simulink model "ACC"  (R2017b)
settings: Solver=FixedStepDiscrete  StartTime=0.0  StopTime=10.0  FixedStep=0.01  RelTol=1e-3  EnableMultiTasking=on
undefined symbols (not defined in the file): ACC_CONST0_NUMB, ACC_CONST1000_NUMB, ACC_CONST100_NUMB, ACC_CONST121_NUMB, ACC_CONST1_NUMB, ACC_CONST2047_NUMB, ACC_CONST60000_NUMB, ACC_CONST60_NUMB, ACC_CONSTF1_NUMB, ACC_RUNTIME_MS, ASWTYPE_FALSE, ASWTYPE_TRUE, CcACC_ACChrgDispSOCPrmt_pct, CcACC_ACChrgMismatch_ms, CcACC_ACChrgPACKVolLim_V, CcACC_ACChrgPACKVolLimTi_ms, CcACC_ACChrgPrmtObcFltLvl_numb, CcACC_ACChrgPrmtVcuFltLvl_numb, CcACC_ACChrgStepCurr_A, CcACC_ACChrgTempPrmtDelayTime_ms, CcACC_ACCrntUnctrolTi_ms, CcACC_ACFullChrgHysVolt_mV, CcACC_ACFullStepChrgTi1_ms, CcACC_ACFullStepChrgTi2_ms, CcACC_ACMaxChrgCurr_A, CcACC_ACStepChrgWaitTime_ms, CcACC_ACStop2DefaultTi_ms, CcACC_ACStop2DefaultTiDelay_ms, CcACC_BatFullResetTime_ms, CcACC_ChrgCrnt0HysVolt_mV, CcACC_ChrgEndDeviationVol1_mV, CcACC_ChrgEndDeviationVol2_mV, CcACC_ChrgEndDeviationVol3_mV, CcACC_ChrgMaxPackVoltLimt_V, CcACC_ChrgPwr1_W, CcACC_ChrgPwr2_W, CcACC_ChrgPwr3_W, CcACC_ChrgSt2StepChrgDeviVol_mV, CcACC_ChrgSt2StepChrgTime_ms, CcACC_ChrgStCutoffTime_ms, CcACC_ChrgStFullChrgCrnt_A, CcACC_CPDutyLowThrhd_pct, CcACC_CrntFilterTi1_cnt, CcACC_CrntFilterTi2_cnt, CcACC_CrntFilterTi2_ms, CcACC_CurrObcPreHeatLowThrhd_A, CcACC_DiffACChrgCrnt_A, CcACC_DiffACChrgCrntTi_ms, CcACC_DispSOCCalStart_pct, CcACC_DispSOCDiff_pct, CcACC_ElecLckRemTimeHold_ms, CcACC_HeatChrgCrnt0Time_ms, CcACC_HeatChrgCrnt1Time_ms, CcACC_Initial500Ti_ms, CcACC_Initial700Ti_ms, CcACC_MaxACChrgCellTemp_C, CcACC_MaxPackVoltLimt_V, CcACC_MinACChrgCellTemp_C, CcACC_MinACChrgCrntRqst_A, CcACC_OBCChrgPwr_W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
libraries: AIWAYS_Powertrain_BMS_lib x94, simulink x2
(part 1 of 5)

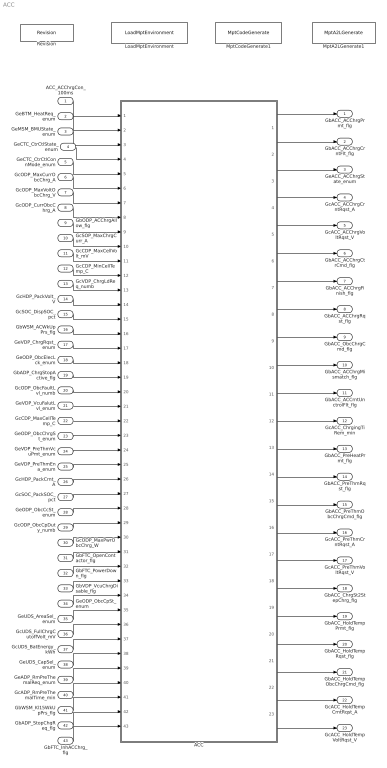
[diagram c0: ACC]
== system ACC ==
  ACC_ACChrgCon_100ms : Inport
  GeBTM_HeatReq_enum : Inport  Port=2
  GeMSM_BMUState_enum : Inport  Port=3
  GeCTC_CtrCtlState_enum : Inport  Port=4
  GeCTC_CtrCtlConnMode_enum : Inport  Port=5
  GcODP_MaxCurrObcChrg_A : Inport  Port=6
  GcODP_MaxVoltObcChrg_V : Inport  Port=7
  GcODP_CurrObcChrg_A : Inport  Port=8
  GbODP_ACChrgAllow_flg : Inport  Port=9
  GcSOP_MaxChrgCurr_A : Inport  Port=10
  GcCDP_MaxCellVolt_mV : Inport  Port=11
  GcCDP_MinCellTemp_C : Inport  Port=12
  GcVDP_ChrgLdReq_numb : Inport  Port=13
  GcHDP_PackVolt_V : Inport  Port=14
  GcSOC_DispSOC_pct : Inport  Port=15
  GbWSM_ACWkUpPrs_flg : Inport  Port=16
  GeVDP_ChrgRqst_enum : Inport  Port=17
  GeODP_ObcElecLck_enum : Inport  Port=18
  GbADP_ChrgStopActive_flg : Inport  Port=19
  GcODP_ObcFaultLvl_numb : Inport  Port=20
  GeVDP_VcuFalutLvl_enum : Inport  Port=21
  GcCDP_MaxCellTemp_C : Inport  Port=22
  GeODP_ObcChrgSt_enum : Inport  Port=23
  GeVDP_PreThmVcuPmt_enum : Inport  Port=24
  GeVDP_PreThmEna_enum : Inport  Port=25
  GcHDP_PackCrnt_A : Inport  Port=26
  GcSOC_PackSOC_pct : Inport  Port=27
  GeODP_ObcCcSt_enum : Inport  Port=28
  GcODP_ObcCpDuty_numb : Inport  Port=29
  GcODP_MaxPwrObcChrg_W : Inport  Port=30
  GbFTC_OpenContactor_flg : Inport  Port=31
  GbFTC_PowerDown_flg : Inport  Port=32
  GbVDP_VcuChrgDisable_flg : Inport  Port=33
  GeODP_ObcCpSt_enum : Inport  Port=34
  GeUDS_AreaSel_enum : Inport  Port=35
  GcUDS_FullChrgCutoffVolt_mV : Inport  Port=36
  GcUDS_BatEnergy_kWh : Inport  Port=37
  GeUDS_CapSel_enum : Inport  Port=38
  GeADP_RmPreThemalReq_enum : Inport  Port=39
  GcADP_RmPreThemalTime_min : Inport  Port=40
  GbWSM_Kl15WkUpPrs_flg : Inport  Port=41
  GbADP_StopChgReq_flg : Inport  Port=42
  GbFTC_InhACChrg_flg : Inport  Port=43
  ACC : Subsystem
  LoadMptEnvironment : AIWAYS_Powertrain_BMS_lib/Config/LoadMptEnvironment  ProjectName=Comm  SuppierID=NewPlatformUAES
  MptA2LGenerate1 : AIWAYS_Powertrain_BMS_lib/Config/MptA2LGenerate  SystemSampleTime=-1
  MptCodeGenerate1 : AIWAYS_Powertrain_BMS_lib/Config/MptCodeGenerate  SystemSampleTime=-1
  Revision : AIWAYS_Powertrain_BMS_lib/Config/Revision  curVersion='M106C108'  newVersion='M106C108'
  GbACC_ACChrgPrmt_flg : Outport
  GbACC_ACChrgCrntFlt_flg : Outport  Port=2
  GeACC_ACChrgState_enum : Outport  Port=3
  GcACC_ACChrgCrntRqst_A : Outport  Port=4
  GcACC_ACChrgVoltRqst_V : Outport  Port=5
  GbACC_ACChrgCtrCmd_flg : Outport  Port=6
  GbACC_ACChrgFinish_flg : Outport  Port=7
  GbACC_ACChrgRqst_flg : Outport  Port=8
  GbACC_ObcChrgCmd_flg : Outport  Port=9
  GbACC_ACChrgMismatch_flg : Outport  Port=10
  GbACC_ACCrntUnctrolFlt_flg : Outport  Port=11
  GcACC_ChrgingTiRem_min : Outport  Port=12
  GbACC_PreHeatPrmt_flg : Outport  Port=13
  GbACC_PreThmRqst_flg : Outport  Port=14
  GbACC_PreThmObcChrgCmd_flg : Outport  Port=15
  GcACC_PreThmCrntRqst_A : Outport  Port=16
  GcACC_PreThmVoltRqst_V : Outport  Port=17
  GbACC_ChrgSt2StepChrg_flg : Outport  Port=18
  GbACC_HoldTempPrmt_flg : Outport  Port=19
  GbACC_HoldTempRqst_flg : Outport  Port=20
  GbACC_HoldTempObcChrgCmd_flg : Outport  Port=21
  GcACC_HoldTempCrntRqst_A : Outport  Port=22
  GcACC_HoldTempVoltRqst_V : Outport  Port=23
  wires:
  ACC_ACChrgCon_100ms/1 -> ACC/1(ACC_ACChrgCon_100ms)
  GeBTM_HeatReq_enum/1 -> ACC/2(GeBTM_HeatReq_enum)
  GeMSM_BMUState_enum/1 -> ACC/3(GeMSM_BMUState_enum)
  GeCTC_CtrCtlState_enum/1 -> ACC/4(GeCTC_CtrCtlState_enum)
  GeCTC_CtrCtlConnMode_enum/1 -> ACC/5(GeCTC_CtrCtlConnMode_enum)
  GcODP_MaxCurrObcChrg_A/1 -> ACC/6(GcODP_MaxCurrObcChrg_A)
  GcODP_MaxVoltObcChrg_V/1 -> ACC/7(GcODP_MaxVoltObcChrg_V)
  GcODP_CurrObcChrg_A/1 -> ACC/8(GcODP_CurrObcChrg_A)
  GbODP_ACChrgAllow_flg/1 -> ACC/9(GbODP_ACChrgAllow_flg)
  GcSOP_MaxChrgCurr_A/1 -> ACC/10(GcSOP_MaxChrgCurr_A)
  GcCDP_MaxCellVolt_mV/1 -> ACC/11(GcCDP_MaxCellVolt_mV)
  GcCDP_MinCellTemp_C/1 -> ACC/12(GcCDP_MinCellTemp_C)
  GcVDP_ChrgLdReq_numb/1 -> ACC/13(GcVDP_ChrgLdReq_numb)
  GcHDP_PackVolt_V/1 -> ACC/14(GcHDP_PackVolt_V)
  GcSOC_DispSOC_pct/1 -> ACC/15(GcSOC_DispSOC_pct)
  GbWSM_ACWkUpPrs_flg/1 -> ACC/16(GbWSM_ACWkUpPrs_flg)
  GeVDP_ChrgRqst_enum/1 -> ACC/17(GeVDP_ChrgRqst_enum)
  GeODP_ObcElecLck_enum/1 -> ACC/18(GeODP_ObcElecLck_enum)
  ACC/1(GbACC_ACChrgPrmt_flg) -> GbACC_ACChrgPrmt_flg/1
  ACC/2(GbACC_ACChrgCrntFlt_flg) -> GbACC_ACChrgCrntFlt_flg/1
  ACC/3(GeACC_ACChrgState_enum) -> GeACC_ACChrgState_enum/1
  ACC/4(GcACC_ACChrgCrntRqst_A) -> GcACC_ACChrgCrntRqst_A/1
  ACC/5(GcACC_ACChrgVoltRqst_V) -> GcACC_ACChrgVoltRqst_V/1
  ACC/6(GbACC_ACChrgCtrCmd_flg) -> GbACC_ACChrgCtrCmd_flg/1
  ACC/7(GbACC_ACChrgFinish_flg) -> GbACC_ACChrgFinish_flg/1
  ACC/8(GbACC_ACChrgRqst_flg) -> GbACC_ACChrgRqst_flg/1
  ACC/9(GbACC_ObcChrgCmd_flg) -> GbACC_ObcChrgCmd_flg/1
  ACC/10(GbACC_ACChrgMismatch_flg) -> GbACC_ACChrgMismatch_flg/1
  ACC/11(GbACC_ACCrntUnctrolFlt_flg) -> GbACC_ACCrntUnctrolFlt_flg/1
  ACC/12(GcACC_ChrgingTiRem_min) -> GcACC_ChrgingTiRem_min/1
  GbADP_ChrgStopActive_flg/1 -> ACC/19(GbADP_ChrgStopActive_flg)
  GeODP_ObcChrgSt_enum/1 -> ACC/23(GeODP_ObcChrgSt_enum)
  GeVDP_VcuFalutLvl_enum/1 -> ACC/21(GeVDP_VcuFalutLvl_enum)
  GcODP_ObcFaultLvl_numb/1 -> ACC/20(GcODP_ObcFaultLvl_numb)
  GcCDP_MaxCellTemp_C/1 -> ACC/22(GcCDP_MaxCellTemp_C)
  ACC/13(GbACC_PreHeatPrmt_flg) -> GbACC_PreHeatPrmt_flg/1
  ACC/14(GbACC_PreThmRqst_flg) -> GbACC_PreThmRqst_flg/1
  GeVDP_PreThmVcuPmt_enum/1 -> ACC/24(GeVDP_PreThmVcuPmt_enum)
  GeVDP_PreThmEna_enum/1 -> ACC/25(GeVDP_PreThmEna_enum)
  ACC/15(GbACC_PreThmObcChrgCmd_flg) -> GbACC_PreThmObcChrgCmd_flg/1
  ACC/16(GcACC_PreThmCrntRqst_A) -> GcACC_PreThmCrntRqst_A/1
  ACC/17(GcACC_PreThmVoltRqst_V) -> GcACC_PreThmVoltRqst_V/1
  GcHDP_PackCrnt_A/1 -> ACC/26(GcHDP_PackCrnt_A)
  GcSOC_PackSOC_pct/1 -> ACC/27(GcSOC_PackSOC_pct)
  GeODP_ObcCcSt_enum/1 -> ACC/28(GeODP_ObcCcSt_enum)
  GcODP_ObcCpDuty_numb/1 -> ACC/29(GcODP_ObcCpDuty_numb)
  GcODP_MaxPwrObcChrg_W/1 -> ACC/30(GcODP_MaxPwrObcChrg_W)
  ACC/18(GbACC_ChrgSt2StepChrg_flg) -> GbACC_ChrgSt2StepChrg_flg/1
  GbFTC_OpenContactor_flg/1 -> ACC/31(GbFTC_OpenContactor_flg)
  GbFTC_PowerDown_flg/1 -> ACC/32(GbFTC_PowerDown_flg)
  GbVDP_VcuChrgDisable_flg/1 -> ACC/33(GbVDP_VcuChrgDisable_flg)
  GeODP_ObcCpSt_enum/1 -> ACC/34(GeODP_ObcCpSt_enum)
  GeUDS_AreaSel_enum/1 -> ACC/35(GeUDS_AreaSel_enum)
  GcUDS_FullChrgCutoffVolt_mV/1 -> ACC/36(GcUDS_FullChrgCutoffVolt_mV)
  GcUDS_BatEnergy_kWh/1 -> ACC/37(GcUDS_BatEnergy_kWh)
  GeUDS_CapSel_enum/1 -> ACC/38(GeUDS_CapSel_enum)
  GeADP_RmPreThemalReq_enum/1 -> ACC/39(GeADP_RmPreThemalReq_enum)
  GcADP_RmPreThemalTime_min/1 -> ACC/40(GcADP_RmPreThemalTime_min)
  GbWSM_Kl15WkUpPrs_flg/1 -> ACC/41(GbWSM_Kl15WkUpPrs_flg)
  ACC/19(GbACC_HoldTempPrmt_flg) -> GbACC_HoldTempPrmt_flg/1
  ACC/20(GbACC_HoldTempRqst_flg) -> GbACC_HoldTempRqst_flg/1
  ACC/21(GbACC_HoldTempObcChrgCmd_flg) -> GbACC_HoldTempObcChrgCmd_flg/1
  ACC/22(GcACC_HoldTempCrntRqst_A) -> GcACC_HoldTempCrntRqst_A/1
  ACC/23(GcACC_HoldTempVoltRqst_V) -> GcACC_HoldTempVoltRqst_V/1
  GbADP_StopChgReq_flg/1 -> ACC/42(GbADP_StopChgReq_flg)
  GbFTC_InhACChrg_flg/1 -> ACC/43(GbFTC_InhACChrg_flg)

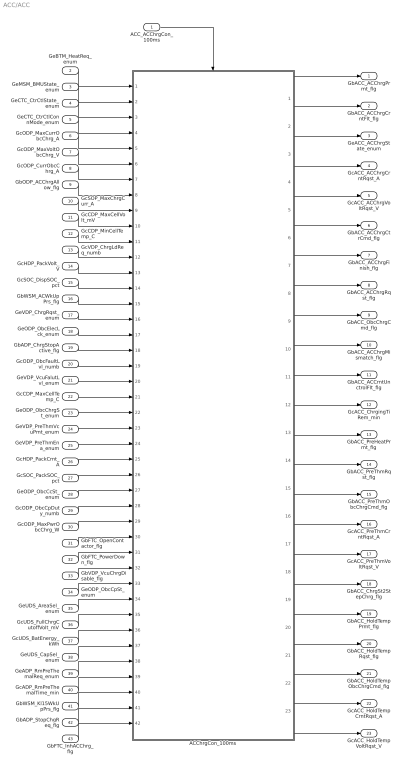
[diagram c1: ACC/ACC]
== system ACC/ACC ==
  ACC_ACChrgCon_100ms : Inport
  GeBTM_HeatReq_enum : Inport  Port=2
  GeMSM_BMUState_enum : Inport  Port=3
  GeCTC_CtrCtlState_enum : Inport  Port=4
  GeCTC_CtrCtlConnMode_enum : Inport  Port=5
  GcODP_MaxCurrObcChrg_A : Inport  Port=6
  GcODP_MaxVoltObcChrg_V : Inport  Port=7
  GcODP_CurrObcChrg_A : Inport  Port=8
  GbODP_ACChrgAllow_flg : Inport  Port=9
  GcSOP_MaxChrgCurr_A : Inport  Port=10
  GcCDP_MaxCellVolt_mV : Inport  Port=11
  GcCDP_MinCellTemp_C : Inport  Port=12
  GcVDP_ChrgLdReq_numb : Inport  Port=13
  GcHDP_PackVolt_V : Inport  Port=14
  GcSOC_DispSOC_pct : Inport  Port=15
  GbWSM_ACWkUpPrs_flg : Inport  Port=16
  GeVDP_ChrgRqst_enum : Inport  Port=17
  GeODP_ObcElecLck_enum : Inport  Port=18
  GbADP_ChrgStopActive_flg : Inport  Port=19
  GcODP_ObcFaultLvl_numb : Inport  Port=20
  GeVDP_VcuFalutLvl_enum : Inport  Port=21
  GcCDP_MaxCellTemp_C : Inport  Port=22
  GeODP_ObcChrgSt_enum : Inport  Port=23
  GeVDP_PreThmVcuPmt_enum : Inport  Port=24
  GeVDP_PreThmEna_enum : Inport  Port=25
  GcHDP_PackCrnt_A : Inport  Port=26
  GcSOC_PackSOC_pct : Inport  Port=27
  GeODP_ObcCcSt_enum : Inport  Port=28
  GcODP_ObcCpDuty_numb : Inport  Port=29
  GcODP_MaxPwrObcChrg_W : Inport  Port=30
  GbFTC_OpenContactor_flg : Inport  Port=31
  GbFTC_PowerDown_flg : Inport  Port=32
  GbVDP_VcuChrgDisable_flg : Inport  Port=33
  GeODP_ObcCpSt_enum : Inport  Port=34
  GeUDS_AreaSel_enum : Inport  Port=35
  GcUDS_FullChrgCutoffVolt_mV : Inport  Port=36
  GcUDS_BatEnergy_kWh : Inport  Port=37
  GeUDS_CapSel_enum : Inport  Port=38
  GeADP_RmPreThemalReq_enum : Inport  Port=39
  GcADP_RmPreThemalTime_min : Inport  Port=40
  GbWSM_Kl15WkUpPrs_flg : Inport  Port=41
  GbADP_StopChgReq_flg : Inport  Port=42
  GbFTC_InhACChrg_flg : Inport  Port=43
  ACChrgCon_100ms : Subsystem
  GbACC_ACChrgPrmt_flg : Outport
  GbACC_ACChrgCrntFlt_flg : Outport  Port=2
  GeACC_ACChrgState_enum : Outport  Port=3
  GcACC_ACChrgCrntRqst_A : Outport  Port=4
  GcACC_ACChrgVoltRqst_V : Outport  Port=5
  GbACC_ACChrgCtrCmd_flg : Outport  Port=6
  GbACC_ACChrgFinish_flg : Outport  Port=7
  GbACC_ACChrgRqst_flg : Outport  Port=8
  GbACC_ObcChrgCmd_flg : Outport  Port=9
  GbACC_ACChrgMismatch_flg : Outport  Port=10
  GbACC_ACCrntUnctrolFlt_flg : Outport  Port=11
  GcACC_ChrgingTiRem_min : Outport  Port=12
  GbACC_PreHeatPrmt_flg : Outport  Port=13
  GbACC_PreThmRqst_flg : Outport  Port=14
  GbACC_PreThmObcChrgCmd_flg : Outport  Port=15
  GcACC_PreThmCrntRqst_A : Outport  Port=16
  GcACC_PreThmVoltRqst_V : Outport  Port=17
  GbACC_ChrgSt2StepChrg_flg : Outport  Port=18
  GbACC_HoldTempPrmt_flg : Outport  Port=19
  GbACC_HoldTempRqst_flg : Outport  Port=20
  GbACC_HoldTempObcChrgCmd_flg : Outport  Port=21
  GcACC_HoldTempCrntRqst_A : Outport  Port=22
  GcACC_HoldTempVoltRqst_V : Outport  Port=23
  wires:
  ACC_ACChrgCon_100ms/1 -> ACChrgCon_100ms/Trigger
  GeBTM_HeatReq_enum/1 -> ACChrgCon_100ms/1(GeBTM_HeatReq_enum)
  GeMSM_BMUState_enum/1 -> ACChrgCon_100ms/2(GeMSM_BMUState_enum)
  GeCTC_CtrCtlState_enum/1 -> ACChrgCon_100ms/3(GeCTC_CtrCtlState_enum)
  GeCTC_CtrCtlConnMode_enum/1 -> ACChrgCon_100ms/4(GeCTC_CtrCtlConnMode_enum)
  GcODP_MaxCurrObcChrg_A/1 -> ACChrgCon_100ms/5(GcODP_MaxCurrObcChrg_A)
  GcODP_MaxVoltObcChrg_V/1 -> ACChrgCon_100ms/6(GcODP_MaxVoltObcChrg_V)
  GcODP_CurrObcChrg_A/1 -> ACChrgCon_100ms/7(GcODP_CurrObcChrg_A)
  GbODP_ACChrgAllow_flg/1 -> ACChrgCon_100ms/8(GbODP_ACChrgAllow_flg)
  GcSOP_MaxChrgCurr_A/1 -> ACChrgCon_100ms/9(GcSOP_MaxChrgCurr_A)
  GcCDP_MaxCellVolt_mV/1 -> ACChrgCon_100ms/10(GcCDP_MaxCellVolt_mV)
  GcCDP_MinCellTemp_C/1 -> ACChrgCon_100ms/11(GcCDP_MinCellTemp_C)
  GcVDP_ChrgLdReq_numb/1 -> ACChrgCon_100ms/12(GcVDP_ChrgLdReq_numb)
  GcHDP_PackVolt_V/1 -> ACChrgCon_100ms/13(GcHDP_PackVolt_V)
  GcSOC_DispSOC_pct/1 -> ACChrgCon_100ms/14(GcSOC_DispSOC_pct)
  GbWSM_ACWkUpPrs_flg/1 -> ACChrgCon_100ms/15(GbWSM_ACWkUpPrs_flg)
  GeVDP_ChrgRqst_enum/1 -> ACChrgCon_100ms/16(GeVDP_ChrgRqst_enum)
  GeODP_ObcElecLck_enum/1 -> ACChrgCon_100ms/17(GeODP_ObcElecLck_enum)
  ACChrgCon_100ms/1(GbACC_ACChrgPrmt_flg) -> GbACC_ACChrgPrmt_flg/1
  ACChrgCon_100ms/2(GbACC_ACChrgCrntFlt_flg) -> GbACC_ACChrgCrntFlt_flg/1
  ACChrgCon_100ms/3(GeACC_ACChrgState_enum) -> GeACC_ACChrgState_enum/1
  ACChrgCon_100ms/4(GcACC_ACChrgCrntRqst_A) -> GcACC_ACChrgCrntRqst_A/1
  ACChrgCon_100ms/5(GcACC_ACChrgVoltRqst_V) -> GcACC_ACChrgVoltRqst_V/1
  ACChrgCon_100ms/6(GbACC_ACChrgCtrCmd_flg) -> GbACC_ACChrgCtrCmd_flg/1
  ACChrgCon_100ms/7(GbACC_ACChrgFinish_flg) -> GbACC_ACChrgFinish_flg/1
  ACChrgCon_100ms/8(GbACC_ACChrgRqst_flg) -> GbACC_ACChrgRqst_flg/1
  ACChrgCon_100ms/9(GbACC_ObcChrgCmd_flg) -> GbACC_ObcChrgCmd_flg/1
  ACChrgCon_100ms/10(GbACC_ACChrgMismatch_flg) -> GbACC_ACChrgMismatch_flg/1
  ACChrgCon_100ms/11(GbACC_ACCrntUnctrolFlt_flg) -> GbACC_ACCrntUnctrolFlt_flg/1
  ACChrgCon_100ms/12(GcACC_ChrgingTiRem_min) -> GcACC_ChrgingTiRem_min/1
  GbADP_ChrgStopActive_flg/1 -> ACChrgCon_100ms/18(GbADP_ChrgStopActive_flg)
  GcODP_ObcFaultLvl_numb/1 -> ACChrgCon_100ms/19(GcODP_ObcFaultLvl_numb)
  GeVDP_VcuFalutLvl_enum/1 -> ACChrgCon_100ms/20(GeVDP_VcuFalutLvl_enum)
  GcCDP_MaxCellTemp_C/1 -> ACChrgCon_100ms/21(GcCDP_MaxCellTemp_C)
  GeODP_ObcChrgSt_enum/1 -> ACChrgCon_100ms/22(GeODP_ObcChrgSt_enum)
  GeVDP_PreThmVcuPmt_enum/1 -> ACChrgCon_100ms/23(GeVDP_PreThmVcuPmt_enum)
  GeVDP_PreThmEna_enum/1 -> ACChrgCon_100ms/24(GeVDP_PreThmEna_enum)
  ACChrgCon_100ms/13(GbACC_PreHeatPrmt_flg) -> GbACC_PreHeatPrmt_flg/1
  ACChrgCon_100ms/14(GbACC_PreThmRqst_flg) -> GbACC_PreThmRqst_flg/1
  ACChrgCon_100ms/15(GbACC_PreThmObcChrgCmd_flg) -> GbACC_PreThmObcChrgCmd_flg/1
  ACChrgCon_100ms/16(GcACC_PreThmCrntRqst_A) -> GcACC_PreThmCrntRqst_A/1
  ACChrgCon_100ms/17(GcACC_PreThmVoltRqst_V) -> GcACC_PreThmVoltRqst_V/1
  GcHDP_PackCrnt_A/1 -> ACChrgCon_100ms/25(GcHDP_PackCrnt_A)
  GcSOC_PackSOC_pct/1 -> ACChrgCon_100ms/26(GcSOC_PackSOC_pct)
  GeODP_ObcCcSt_enum/1 -> ACChrgCon_100ms/27(GeODP_ObcCcSt_enum)
  GcODP_ObcCpDuty_numb/1 -> ACChrgCon_100ms/28(GcODP_ObcCpDuty_numb)
  GcODP_MaxPwrObcChrg_W/1 -> ACChrgCon_100ms/29(GcODP_MaxPwrObcChrg_W)
  ACChrgCon_100ms/18(GbACC_ChrgSt2StepChrg_flg) -> GbACC_ChrgSt2StepChrg_flg/1
  GbFTC_OpenContactor_flg/1 -> ACChrgCon_100ms/30(GbFTC_OpenContactor_flg)
  GbFTC_PowerDown_flg/1 -> ACChrgCon_100ms/31(GbFTC_PowerDown_flg)
  GbVDP_VcuChrgDisable_flg/1 -> ACChrgCon_100ms/32(GbVDP_VcuChrgDisable_flg)
  GeODP_ObcCpSt_enum/1 -> ACChrgCon_100ms/33(GeODP_ObcCpSt_enum)
  GeUDS_AreaSel_enum/1 -> ACChrgCon_100ms/34(GeUDS_AreaSel_enum)
  GcUDS_FullChrgCutoffVolt_mV/1 -> ACChrgCon_100ms/35(GcUDS_FullChrgCutoffVolt_mV)
  GcUDS_BatEnergy_kWh/1 -> ACChrgCon_100ms/36(GcUDS_BatEnergy_kWh)
  GeUDS_CapSel_enum/1 -> ACChrgCon_100ms/37(GeUDS_CapSel_enum)
  ACChrgCon_100ms/19(GbACC_HoldTempPrmt_flg) -> GbACC_HoldTempPrmt_flg/1
  ACChrgCon_100ms/20(GbACC_HoldTempRqst_flg) -> GbACC_HoldTempRqst_flg/1
  ACChrgCon_100ms/21(GbACC_HoldTempObcChrgCmd_flg) -> GbACC_HoldTempObcChrgCmd_flg/1
  ACChrgCon_100ms/22(GcACC_HoldTempCrntRqst_A) -> GcACC_HoldTempCrntRqst_A/1
  ACChrgCon_100ms/23(GcACC_HoldTempVoltRqst_V) -> GcACC_HoldTempVoltRqst_V/1
  GeADP_RmPreThemalReq_enum/1 -> ACChrgCon_100ms/38(GeADP_RmPreThemalReq_enum)
  GcADP_RmPreThemalTime_min/1 -> ACChrgCon_100ms/39(GcADP_RmPreThemalTime_min)
  GbWSM_Kl15WkUpPrs_flg/1 -> ACChrgCon_100ms/40(GbWSM_Kl15WkUpPrs_flg)
  GbADP_StopChgReq_flg/1 -> ACChrgCon_100ms/41(GbADP_StopChgReq_flg)
  GbFTC_InhACChrg_flg/1 -> ACChrgCon_100ms/42(GbFTC_InhACChrg_flg)

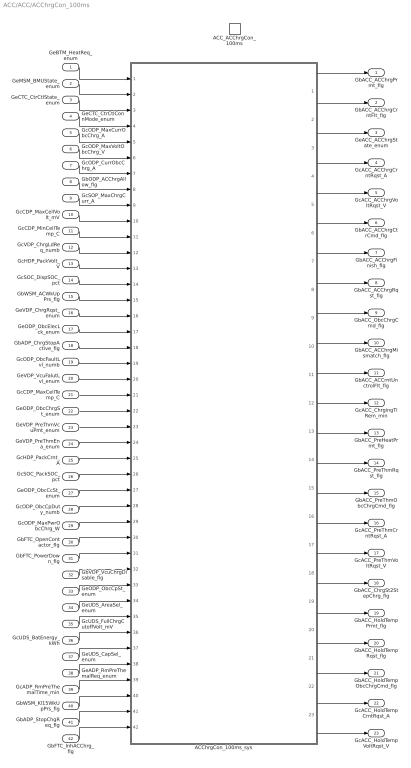
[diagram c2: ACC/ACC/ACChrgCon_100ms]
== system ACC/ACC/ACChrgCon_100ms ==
  GeBTM_HeatReq_enum : Inport
  GeMSM_BMUState_enum : Inport  Port=2
  GeCTC_CtrCtlState_enum : Inport  Port=3
  GeCTC_CtrCtlConnMode_enum : Inport  Port=4
  GcODP_MaxCurrObcChrg_A : Inport  Port=5
  GcODP_MaxVoltObcChrg_V : Inport  Port=6
  GcODP_CurrObcChrg_A : Inport  Port=7
  GbODP_ACChrgAllow_flg : Inport  Port=8
  GcSOP_MaxChrgCurr_A : Inport  Port=9
  GcCDP_MaxCellVolt_mV : Inport  Port=10
  GcCDP_MinCellTemp_C : Inport  Port=11
  GcVDP_ChrgLdReq_numb : Inport  Port=12
  GcHDP_PackVolt_V : Inport  Port=13
  GcSOC_DispSOC_pct : Inport  Port=14
  GbWSM_ACWkUpPrs_flg : Inport  Port=15
  GeVDP_ChrgRqst_enum : Inport  Port=16
  GeODP_ObcElecLck_enum : Inport  Port=17
  GbADP_ChrgStopActive_flg : Inport  Port=18
  GcODP_ObcFaultLvl_numb : Inport  Port=19
  GeVDP_VcuFalutLvl_enum : Inport  Port=20
  GcCDP_MaxCellTemp_C : Inport  Port=21
  GeODP_ObcChrgSt_enum : Inport  Port=22
  GeVDP_PreThmVcuPmt_enum : Inport  Port=23
  GeVDP_PreThmEna_enum : Inport  Port=24
  GcHDP_PackCrnt_A : Inport  Port=25
  GcSOC_PackSOC_pct : Inport  Port=26
  GeODP_ObcCcSt_enum : Inport  Port=27
  GcODP_ObcCpDuty_numb : Inport  Port=28
  GcODP_MaxPwrObcChrg_W : Inport  Port=29
  GbFTC_OpenContactor_flg : Inport  Port=30
  GbFTC_PowerDown_flg : Inport  Port=31
  GbVDP_VcuChrgDisable_flg : Inport  Port=32
  GeODP_ObcCpSt_enum : Inport  Port=33
  GeUDS_AreaSel_enum : Inport  Port=34
  GcUDS_FullChrgCutoffVolt_mV : Inport  Port=35
  GcUDS_BatEnergy_kWh : Inport  Port=36
  GeUDS_CapSel_enum : Inport  Port=37
  GeADP_RmPreThemalReq_enum : Inport  Port=38
  GcADP_RmPreThemalTime_min : Inport  Port=39
  GbWSM_Kl15WkUpPrs_flg : Inport  Port=40
  GbADP_StopChgReq_flg : Inport  Port=41
  GbFTC_InhACChrg_flg : Inport  Port=42
  ACC_ACChrgCon_100ms : TriggerPort  TriggerType=function-call  VariantControl=(inherit)
  ACChrgCon_100ms_sys : Subsystem
  GbACC_ACChrgPrmt_flg : Outport
  GbACC_ACChrgCrntFlt_flg : Outport  Port=2
  GeACC_ACChrgState_enum : Outport  Port=3
  GcACC_ACChrgCrntRqst_A : Outport  Port=4
  GcACC_ACChrgVoltRqst_V : Outport  Port=5
  GbACC_ACChrgCtrCmd_flg : Outport  Port=6
  GbACC_ACChrgFinish_flg : Outport  Port=7
  GbACC_ACChrgRqst_flg : Outport  Port=8
  GbACC_ObcChrgCmd_flg : Outport  Port=9
  GbACC_ACChrgMismatch_flg : Outport  Port=10
  GbACC_ACCrntUnctrolFlt_flg : Outport  Port=11
  GcACC_ChrgingTiRem_min : Outport  Port=12
  GbACC_PreHeatPrmt_flg : Outport  Port=13
  GbACC_PreThmRqst_flg : Outport  Port=14
  GbACC_PreThmObcChrgCmd_flg : Outport  Port=15
  GcACC_PreThmCrntRqst_A : Outport  Port=16
  GcACC_PreThmVoltRqst_V : Outport  Port=17
  GbACC_ChrgSt2StepChrg_flg : Outport  Port=18
  GbACC_HoldTempPrmt_flg : Outport  Port=19
  GbACC_HoldTempRqst_flg : Outport  Port=20
  GbACC_HoldTempObcChrgCmd_flg : Outport  Port=21
  GcACC_HoldTempCrntRqst_A : Outport  Port=22
  GcACC_HoldTempVoltRqst_V : Outport  Port=23
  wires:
  GeBTM_HeatReq_enum/1 -> ACChrgCon_100ms_sys/1(GeBTM_HeatReq_enum)
  GeMSM_BMUState_enum/1 -> ACChrgCon_100ms_sys/2(GeMSM_BMUState_enum)
  GeCTC_CtrCtlState_enum/1 -> ACChrgCon_100ms_sys/3(GeCTC_CtrCtlState_enum)
  GeCTC_CtrCtlConnMode_enum/1 -> ACChrgCon_100ms_sys/4(GeCTC_CtrCtlConnMode_enum)
  GcODP_MaxCurrObcChrg_A/1 -> ACChrgCon_100ms_sys/5(GcODP_MaxCurrObcChrg_A)
  GcODP_MaxVoltObcChrg_V/1 -> ACChrgCon_100ms_sys/6(GcODP_MaxVoltObcChrg_V)
  GcODP_CurrObcChrg_A/1 -> ACChrgCon_100ms_sys/7(GcODP_CurrObcChrg_A)
  GbODP_ACChrgAllow_flg/1 -> ACChrgCon_100ms_sys/8(GbODP_ACChrgAllow_flg)
  GcSOP_MaxChrgCurr_A/1 -> ACChrgCon_100ms_sys/9(GcSOP_MaxChrgCurr_A)
  GcCDP_MaxCellVolt_mV/1 -> ACChrgCon_100ms_sys/10(GcCDP_MaxCellVolt_mV)
  GcCDP_MinCellTemp_C/1 -> ACChrgCon_100ms_sys/11(GcCDP_MinCellTemp_C)
  GcVDP_ChrgLdReq_numb/1 -> ACChrgCon_100ms_sys/12(GcVDP_ChrgLdReq_numb)
  GcHDP_PackVolt_V/1 -> ACChrgCon_100ms_sys/13(GcHDP_PackVolt_V)
  GcSOC_DispSOC_pct/1 -> ACChrgCon_100ms_sys/14(GcSOC_DispSOC_pct)
  GbWSM_ACWkUpPrs_flg/1 -> ACChrgCon_100ms_sys/15(GbWSM_ACWkUpPrs_flg)
  GeVDP_ChrgRqst_enum/1 -> ACChrgCon_100ms_sys/16(GeVDP_ChrgRqst_enum)
  GeODP_ObcElecLck_enum/1 -> ACChrgCon_100ms_sys/17(GeODP_ObcElecLck_enum)
  ACChrgCon_100ms_sys/1(GbACC_ACChrgPrmt_flg) -> GbACC_ACChrgPrmt_flg/1
  ACChrgCon_100ms_sys/2(GbACC_ACChrgCrntFlt_flg) -> GbACC_ACChrgCrntFlt_flg/1
  ACChrgCon_100ms_sys/3(GeACC_ACChrgState_enum) -> GeACC_ACChrgState_enum/1
  ACChrgCon_100ms_sys/4(GcACC_ACChrgCrntRqst_A) -> GcACC_ACChrgCrntRqst_A/1
  ACChrgCon_100ms_sys/5(GcACC_ACChrgVoltRqst_V) -> GcACC_ACChrgVoltRqst_V/1
  ACChrgCon_100ms_sys/6(GbACC_ACChrgCtrCmd_flg) -> GbACC_ACChrgCtrCmd_flg/1
  ACChrgCon_100ms_sys/7(GbACC_ACChrgFinish_flg) -> GbACC_ACChrgFinish_flg/1
  ACChrgCon_100ms_sys/8(GbACC_ACChrgRqst_flg) -> GbACC_ACChrgRqst_flg/1
  ACChrgCon_100ms_sys/9(GbACC_ObcChrgCmd_flg) -> GbACC_ObcChrgCmd_flg/1
  ACChrgCon_100ms_sys/10(GbACC_ACChrgMismatch_flg) -> GbACC_ACChrgMismatch_flg/1
  ACChrgCon_100ms_sys/11(GbACC_ACCrntUnctrolFlt_flg) -> GbACC_ACCrntUnctrolFlt_flg/1
  ACChrgCon_100ms_sys/12(GcACC_ChrgingTiRem_min) -> GcACC_ChrgingTiRem_min/1
  GbADP_ChrgStopActive_flg/1 -> ACChrgCon_100ms_sys/18(GbADP_ChrgStopActive_flg)
  GcODP_ObcFaultLvl_numb/1 -> ACChrgCon_100ms_sys/19(GcODP_ObcFaultLvl_numb)
  GeVDP_VcuFalutLvl_enum/1 -> ACChrgCon_100ms_sys/20(GeVDP_VcuFalutLvl_enum)
  GcCDP_MaxCellTemp_C/1 -> ACChrgCon_100ms_sys/21(GcCDP_MaxCellTemp_C)
  GeODP_ObcChrgSt_enum/1 -> ACChrgCon_100ms_sys/22(GeODP_ObcChrgSt_enum)
  GeVDP_PreThmVcuPmt_enum/1 -> ACChrgCon_100ms_sys/23(GeVDP_PreThmVcuPmt_enum)
  GeVDP_PreThmEna_enum/1 -> ACChrgCon_100ms_sys/24(GeVDP_PreThmEna_enum)
  ACChrgCon_100ms_sys/13(GbACC_PreHeatPrmt_flg) -> GbACC_PreHeatPrmt_flg/1
  ACChrgCon_100ms_sys/14(GbACC_PreThmRqst_flg) -> GbACC_PreThmRqst_flg/1
  ACChrgCon_100ms_sys/15(GbACC_PreThmObcChrgCmd_flg) -> GbACC_PreThmObcChrgCmd_flg/1
  ACChrgCon_100ms_sys/16(GcACC_PreThmCrntRqst_A) -> GcACC_PreThmCrntRqst_A/1
  ACChrgCon_100ms_sys/17(GcACC_PreThmVoltRqst_V) -> GcACC_PreThmVoltRqst_V/1
  GcHDP_PackCrnt_A/1 -> ACChrgCon_100ms_sys/25(GcHDP_PackCrnt_A)
  GcSOC_PackSOC_pct/1 -> ACChrgCon_100ms_sys/26(GcSOC_PackSOC_pct)
  GeODP_ObcCcSt_enum/1 -> ACChrgCon_100ms_sys/27(GeODP_ObcCcSt_enum)
  GcODP_ObcCpDuty_numb/1 -> ACChrgCon_100ms_sys/28(GcODP_ObcCpDuty_numb)
  GcODP_MaxPwrObcChrg_W/1 -> ACChrgCon_100ms_sys/29(GcODP_MaxPwrObcChrg_W)
  ACChrgCon_100ms_sys/18(GbACC_ChrgSt2StepChrg_flg) -> GbACC_ChrgSt2StepChrg_flg/1
  GbFTC_OpenContactor_flg/1 -> ACChrgCon_100ms_sys/30(GbFTC_OpenContactor_flg)
  GbFTC_PowerDown_flg/1 -> ACChrgCon_100ms_sys/31(GbFTC_PowerDown_flg)
  GbVDP_VcuChrgDisable_flg/1 -> ACChrgCon_100ms_sys/32(GbVDP_VcuChrgDisable_flg)
  GeODP_ObcCpSt_enum/1 -> ACChrgCon_100ms_sys/33(GeODP_ObcCpSt_enum)
  GeUDS_AreaSel_enum/1 -> ACChrgCon_100ms_sys/34(GeUDS_AreaSel_enum)
  GcUDS_FullChrgCutoffVolt_mV/1 -> ACChrgCon_100ms_sys/35(GcUDS_FullChrgCutoffVolt_mV)
  GcUDS_BatEnergy_kWh/1 -> ACChrgCon_100ms_sys/36(GcUDS_BatEnergy_kWh)
  GeUDS_CapSel_enum/1 -> ACChrgCon_100ms_sys/37(GeUDS_CapSel_enum)
  GeADP_RmPreThemalReq_enum/1 -> ACChrgCon_100ms_sys/38(GeADP_RmPreThemalReq_enum)
  GcADP_RmPreThemalTime_min/1 -> ACChrgCon_100ms_sys/39(GcADP_RmPreThemalTime_min)
  GbWSM_Kl15WkUpPrs_flg/1 -> ACChrgCon_100ms_sys/40(GbWSM_Kl15WkUpPrs_flg)
  ACChrgCon_100ms_sys/19(GbACC_HoldTempPrmt_flg) -> GbACC_HoldTempPrmt_flg/1
  ACChrgCon_100ms_sys/20(GbACC_HoldTempRqst_flg) -> GbACC_HoldTempRqst_flg/1
  ACChrgCon_100ms_sys/21(GbACC_HoldTempObcChrgCmd_flg) -> GbACC_HoldTempObcChrgCmd_flg/1
  ACChrgCon_100ms_sys/22(GcACC_HoldTempCrntRqst_A) -> GcACC_HoldTempCrntRqst_A/1
  ACChrgCon_100ms_sys/23(GcACC_HoldTempVoltRqst_V) -> GcACC_HoldTempVoltRqst_V/1
  GbADP_StopChgReq_flg/1 -> ACChrgCon_100ms_sys/41(GbADP_StopChgReq_flg)
  GbFTC_InhACChrg_flg/1 -> ACChrgCon_100ms_sys/42(GbFTC_InhACChrg_flg)

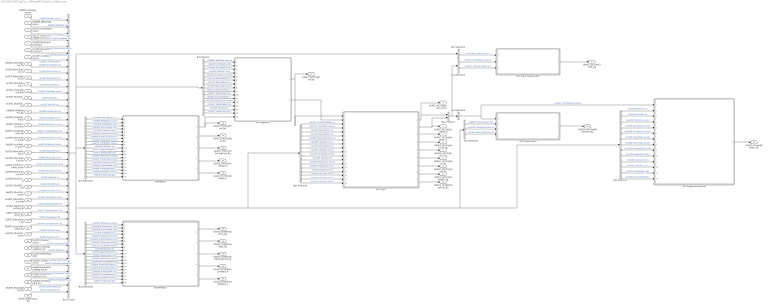
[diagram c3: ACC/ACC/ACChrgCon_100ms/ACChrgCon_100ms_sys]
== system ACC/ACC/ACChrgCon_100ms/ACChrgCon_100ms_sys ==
  GeBTM_HeatReq_enum : Inport
  GeMSM_BMUState_enum : Inport  Port=2
  GeCTC_CtrCtlState_enum : Inport  Port=3
  GeCTC_CtrCtlConnMode_enum : Inport  Port=4
  GcODP_MaxCurrObcChrg_A : Inport  Port=5
  GcODP_MaxVoltObcChrg_V : Inport  Port=6
  GcODP_CurrObcChrg_A : Inport  Port=7
  GbODP_ACChrgAllow_flg : Inport  Port=8
  GcSOP_MaxChrgCurr_A : Inport  Port=9
  GcCDP_MaxCellVolt_mV : Inport  Port=10
  GcCDP_MinCellTemp_C : Inport  Port=11
  GcVDP_ChrgLdReq_numb : Inport  Port=12
  GcHDP_PackVolt_V : Inport  Port=13
  GcSOC_DispSOC_pct : Inport  Port=14
  GbWSM_ACWkUpPrs_flg : Inport  Port=15
  GeVDP_ChrgRqst_enum : Inport  Port=16
  GeODP_ObcElecLck_enum : Inport  Port=17
  GbADP_ChrgStopActive_flg : Inport  Port=18
  GcODP_ObcFaultLvl_numb : Inport  Port=19
  GeVDP_VcuFalutLvl_enum : Inport  Port=20
  GcCDP_MaxCellTemp_C : Inport  Port=21
  GeODP_ObcChrgSt_enum : Inport  Port=22
  GeVDP_PreThmVcuPmt_enum : Inport  Port=23
  GeVDP_PreThmEna_enum : Inport  Port=24
  GcHDP_PackCrnt_A : Inport  Port=25
  GcSOC_PackSOC_pct : Inport  Port=26
  GeODP_ObcCcSt_enum : Inport  Port=27
  GcODP_ObcCpDuty_numb : Inport  Port=28
  GcODP_MaxPwrObcChrg_W : Inport  Port=29
  GbFTC_OpenContactor_flg : Inport  Port=30
  GbFTC_PowerDown_flg : Inport  Port=31
  GbVDP_VcuChrgDisable_flg : Inport  Port=32
  GeODP_ObcCpSt_enum : Inport  Port=33
  GeUDS_AreaSel_enum : Inport  Port=34
  GcUDS_FullChrgCutoffVolt_mV : Inport  Port=35
  GcUDS_BatEnergy_kWh : Inport  Port=36
  GeUDS_CapSel_enum : Inport  Port=37
  GeADP_RmPreThemalReq_enum : Inport  Port=38
  GcADP_RmPreThemalTime_min : Inport  Port=39
  GbWSM_Kl15WkUpPrs_flg : Inport  Port=40
  GbADP_StopChgReq_flg : Inport  Port=41
  GbFTC_InhACChrg_flg : Inport  Port=42
  ACChrgCrntReponseFlt : Subsystem
  ACChrgCtl : Subsystem
  ACChrgMismatch : Subsystem
  ACChrgPermit : Subsystem
  ACChrgRemainingTime : Subsystem
  Bus Creator : BusCreator  Inputs=42
  Bus Creator1 : BusCreator  Inputs=2
  Bus Selector : BusSelector  OutputSignals=GeMSM_BMUState_enum,GbWSM_ACWkUpPrs_flg,GbODP_ACChrgAllow_flg,GcSOC_DispSOC_pct,GeVDP_VcuFalutLvl_enum,GcCDP_MinCellTemp_C,GcCDP_MaxCellTemp_C,GeODP_ObcChrgSt_enum,GbFTC_OpenContactor_flg,GbFTC_PowerDown_flg,GbVDP_VcuChrgDisable_flg,GcODP_ObcFaultLvl_numb,GbADP_StopChgReq_flg,GcHDP_PackVolt_V,GbFTC_InhACChrg_flg
  Bus Selector1 : BusSelector  OutputSignals=GeCTC_CtrCtlConnMode_enum,GeCTC_CtrCtlState_enum,GcSOP_MaxChrgCurr_A,GcCDP_MaxCellVolt_mV,GcODP_MaxCurrObcChrg_A,GeBTM_HeatReq_enum,GcCDP_MinCellTemp_C,GeVDP_ChrgRqst_enum,GcVDP_ChrgLdReq_numb,GcHDP_PackVolt_V,GeODP_ObcElecLck_enum,GbADP_ChrgStopActive_flg,GcSOC_DispSOC_pct,GeODP_ObcCpSt_enum,GeUDS_AreaSel_enum,GcUDS_FullChrgCutoffVolt_mV
  Bus Selector2 : BusSelector  OutputSignals=GcODP_CurrObcChrg_A
  Bus Selector3 : BusSelector  OutputSignals=GeACC_ACChrgState_enum,GcACC_ACChrgCrntRqst_A
  Bus Selector4 : BusSelector  OutputSignals=GeACC_ACChrgState_enum
  Bus Selector5 : BusSelector  OutputSignals=GbODP_ACChrgAllow_flg,GcODP_MaxVoltObcChrg_V,GcODP_MaxCurrObcChrg_A
  Bus Selector6 : BusSelector  OutputSignals=GcCDP_MinCellTemp_C,GeMSM_BMUState_enum,GbWSM_ACWkUpPrs_flg,GbODP_ACChrgAllow_flg,GcSOC_DispSOC_pct,GeVDP_VcuFalutLvl_enum,GeVDP_PreThmVcuPmt_enum,GeODP_ObcChrgSt_enum,GeCTC_CtrCtlState_enum,GcHDP_PackVolt_V,GbFTC_OpenContactor_flg,GbFTC_PowerDown_flg,GcODP_ObcFaultLvl_numb,GeVDP_PreThmEna_enum,GcODP_CurrObcChrg_A,GbADP_StopChgReq_flg,GbADP_ChrgStopActive_flg,GeUDS_AreaSel_enum,GbFTC_InhACChrg_flg
  Bus Selector7 : BusSelector  OutputSignals=GcHDP_PackCrnt_A,GcHDP_PackVolt_V,GeODP_ObcCcSt_enum,GcODP_ObcCpDuty_numb,GeODP_ObcElecLck_enum,GcVDP_ChrgLdReq_numb,GeODP_ObcChrgSt_enum,GcODP_MaxPwrObcChrg_W,GcUDS_BatEnergy_kWh,GeUDS_CapSel_enum,GcSOC_DispSOC_pct,GcCDP_MaxCellVolt_mV,GcUDS_FullChrgCutoffVolt_mV
  Bus Selector8 : BusSelector  OutputSignals=GeMSM_BMUState_enum,GbWSM_ACWkUpPrs_flg,GbODP_ACChrgAllow_flg,GcSOC_DispSOC_pct,GeVDP_VcuFalutLvl_enum,GeVDP_PreThmVcuPmt_enum,GeODP_ObcChrgSt_enum,GeCTC_CtrCtlState_enum,GcHDP_PackVolt_V,GbFTC_OpenContactor_flg,GbFTC_PowerDown_flg,GcODP_ObcFaultLvl_numb,GbWSM_Kl15WkUpPrs_flg,GeADP_RmPreThemalReq_enum,GcADP_RmPreThemalTime_min,GbADP_StopChgReq_flg,GbADP_ChrgStopActive_flg,GeUDS_AreaSel_enum,GbFTC_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
  HoldTempCtl : Subsystem
  PreHeatCtl : Subsystem
  GbACC_ACChrgPrmt_flg : Outport
  GbACC_ACChrgCrntFlt_flg : Outport  Port=2
  GeACC_ACChrgState_enum : Outport  Port=3
  GcACC_ACChrgCrntRqst_A : Outport  Port=4
  GcACC_ACChrgVoltRqst_V : Outport  Port=5
  GbACC_ACChrgCtrCmd_flg : Outport  Port=6
  GbACC_ACChrgFinish_flg : Outport  Port=7
  GbACC_ACChrgRqst_flg : Outport  Port=8
  GbACC_ObcChrgCmd_flg : Outport  Port=9
  GbACC_ACChrgMismatch_flg : Outport  Port=10
  GbACC_ACCrntUnctrolFlt_flg : Outport  Port=11
  GcACC_ChrgingTiRem_min : Outport  Port=12
  GbACC_PreHeatPrmt_flg : Outport  Port=13
  GbACC_PreThmRqst_flg : Outport  Port=14
  GbACC_PreThmObcChrgCmd_flg : Outport  Port=15
  GcACC_PreThmCrntRqst_A : Outport  Port=16
  GcACC_PreThmVoltRqst_V : Outport  Port=17
  GbACC_ChrgSt2StepChrg_flg : Outport  Port=18
  GbACC_HoldTempPrmt_flg : Outport  Port=19
  GbACC_HoldTempRqst_flg : Outport  Port=20
  GbACC_HoldTempObcChrgCmd_flg : Outport  Port=21
  GcACC_HoldTempCrntRqst_A : Outport  Port=22
  GcACC_HoldTempVoltRqst_V : Outport  Port=23
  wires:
  ACChrgPermit/1(GbACC_ACChrgPrmt_flg) -> GbACC_ACChrgPrmt_flg/1, ACChrgCtl/1(GbACC_ACChrgPrmt_flg)
  GeBTM_HeatReq_enum/1 -> Bus Creator/1  "GeBTM_HeatReq_enum"
  GeMSM_BMUState_enum/1 -> Bus Creator/2  "GeMSM_BMUState_enum"
  GeCTC_CtrCtlState_enum/1 -> Bus Creator/3  "GeCTC_CtrCtlState_enum"
  GeCTC_CtrCtlConnMode_enum/1 -> Bus Creator/4  "GeCTC_CtrCtlConnMode_enum"
  GcODP_MaxCurrObcChrg_A/1 -> Bus Creator/5  "GcODP_MaxCurrObcChrg_A"
  GcODP_MaxVoltObcChrg_V/1 -> Bus Creator/6  "GcODP_MaxVoltObcChrg_V"
  GcODP_CurrObcChrg_A/1 -> Bus Creator/7  "GcODP_CurrObcChrg_A"
  GbODP_ACChrgAllow_flg/1 -> Bus Creator/8  "GbODP_ACChrgAllow_flg"
  GcSOP_MaxChrgCurr_A/1 -> Bus Creator/9  "GcSOP_MaxChrgCurr_A"
  GcCDP_MaxCellVolt_mV/1 -> Bus Creator/10  "GcCDP_MaxCellVolt_mV"
  GcCDP_MinCellTemp_C/1 -> Bus Creator/11  "GcCDP_MinCellTemp_C"
  GcVDP_ChrgLdReq_numb/1 -> Bus Creator/12  "GcVDP_ChrgLdReq_numb"
  GcHDP_PackVolt_V/1 -> Bus Creator/13  "GcHDP_PackVolt_V"
  GcSOC_DispSOC_pct/1 -> Bus Creator/14  "GcSOC_DispSOC_pct"
  GbWSM_ACWkUpPrs_flg/1 -> Bus Creator/15  "GbWSM_ACWkUpPrs_flg"
  Bus Creator/1 -> Bus Selector2/1, Bus Selector/1, Bus Selector6/1, Bus Selector8/1, Bus Selector5/1, Bus Selector7/1, Bus Selector1/1
  Bus Selector/1 -> ACChrgPermit/1(GeMSM_BMUState_enum)  "<GeMSM_BMUState_enum>"
  Bus Selector/2 -> ACChrgPermit/2(GbWSM_ACWkUpPrs_flg)  "<GbWSM_ACWkUpPrs_flg>"
  Bus Selector/3 -> ACChrgPermit/3(GbODP_ACChrgAllow_flg)  "<GbODP_ACChrgAllow_flg>"
  Bus Selector/4 -> ACChrgPermit/4(GcSOC_DispSOC_pct)  "<GcSOC_DispSOC_pct>"
  Bus Selector1/1 -> ACChrgCtl/3(GeCTC_CtrCtlConnMode_enum)  "<GeCTC_CtrCtlConnMode_enum>"
  Bus Selector1/2 -> ACChrgCtl/4(GeCTC_CtrCtlState_enum)  "<GeCTC_CtrCtlState_enum>"
  Bus Selector1/3 -> ACChrgCtl/5(GcSOP_MaxChrgCurr_A)  "<GcSOP_MaxChrgCurr_A>"
  Bus Selector1/4 -> ACChrgCtl/6(GcCDP_MaxCellVolt_mV)  "<GcCDP_MaxCellVolt_mV>"
  Bus Selector1/5 -> ACChrgCtl/7(GcODP_MaxCurrObcChrg_A)  "<GcODP_MaxCurrObcChrg_A>"
  Bus Selector1/6 -> ACChrgCtl/8(GeBTM_HeatReq_enum)  "<GeBTM_HeatReq_enum>"
  Bus Selector1/7 -> ACChrgCtl/9(GcCDP_MinCellTemp_C)  "<GcCDP_MinCellTemp_C>"
  GeVDP_ChrgRqst_enum/1 -> Bus Creator/16  "GeVDP_ChrgRqst_enum"
  Bus Selector1/8 -> ACChrgCtl/10(GeVDP_ChrgRqst_enum)  "<GeVDP_ChrgRqst_enum>"
  GeODP_ObcElecLck_enum/1 -> Bus Creator/17  "GeODP_ObcElecLck_enum"
  Bus Selector1/9 -> ACChrgCtl/11(GcVDP_ChrgLdReq_numb)  "<GcVDP_ChrgLdReq_numb>"
  Bus Selector1/10 -> ACChrgCtl/12(GcHDP_PackVolt_V)  "<GcHDP_PackVolt_V>"
  Bus Selector1/11 -> ACChrgCtl/13(GeODP_ObcElecLck_enum)  "<GeODP_ObcElecLck_enum>"
  Bus Selector2/1 -> ACChrgCrntReponseFlt/1(GcODP_CurrObcChrg_A)  "<GcODP_CurrObcChrg_A>"
  ACChrgCrntReponseFlt/1(GbACC_ACChrgCrntFlt_flg) -> GbACC_ACChrgCrntFlt_flg/1
  ACChrgCtl/1(GeACC_ACChrgState_enum) -> GeACC_ACChrgState_enum/1, Bus Creator1/1
  ACChrgCtl/2(GcACC_ACChrgCrntRqst_A) -> Bus Creator1/2, GcACC_ACChrgCrntRqst_A/1
  Bus Creator1/1 -> Bus Selector3/1, Bus Selector4/1
  Bus Selector3/2 -> ACChrgCrntReponseFlt/3(GcACC_ACChrgCrntRqst_A)  "<GcACC_ACChrgCrntRqst_A>"
  Bus Selector3/1 -> ACChrgCrntReponseFlt/2(GeACC_ACChrgState_enum)  "<GeACC_ACChrgState_enum>"
  Bus Selector4/1 -> ACChrgRemainingTime/1(GeACC_ACChrgState_enum), ACChrgMismatch/1(GeACC_ACChrgState_enum)  "<GeACC_ACChrgState_enum>"
  ACChrgCtl/3(GcACC_ACChrgVoltRqst_V) -> GcACC_ACChrgVoltRqst_V/1
  ACChrgCtl/4(GbACC_ACChrgCtrCmd_flg) -> GbACC_ACChrgCtrCmd_flg/1
  ACChrgCtl/5(GbACC_ACChrgFinish_flg) -> GbACC_ACChrgFinish_flg/1
  ACChrgCtl/6(GbACC_ACChrgRqst_flg) -> GbACC_ACChrgRqst_flg/1
  ACChrgCtl/7(GbACC_ObcChrgCmd_flg) -> GbACC_ObcChrgCmd_flg/1
  Bus Selector5/1 -> ACChrgMismatch/2(GbODP_ACChrgAllow_flg)  "<GbODP_ACChrgAllow_flg>"
  ACChrgMismatch/1(GbACC_ACChrgMismatch_flg) -> GbACC_ACChrgMismatch_flg/1
  ACChrgCtl/8(GbACC_ACCrntUnctrolFlt_flg) -> GbACC_ACCrntUnctrolFlt_flg/1
  Bus Selector5/2 -> ACChrgMismatch/3(GcODP_MaxVoltObcChrg_V)  "<GcODP_MaxVoltObcChrg_V>"
  Bus Selector5/3 -> ACChrgMismatch/4(GcODP_MaxCurrObcChrg_A)  "<GcODP_MaxCurrObcChrg_A>"
  ACChrgRemainingTime/1(GcACC_ChrgingTiRem_min) -> GcACC_ChrgingTiRem_min/1
  GbADP_ChrgStopActive_flg/1 -> Bus Creator/18  "GbADP_ChrgStopActive_flg"
  Bus Selector1/12 -> ACChrgCtl/14(GbADP_ChrgStopActive_flg)  "<GbADP_ChrgStopActive_flg>"
  GcODP_ObcFaultLvl_numb/1 -> Bus Creator/19  "GcODP_ObcFaultLvl_numb"
  GeVDP_VcuFalutLvl_enum/1 -> Bus Creator/20  "GeVDP_VcuFalutLvl_enum"
  GcCDP_MaxCellTemp_C/1 -> Bus Creator/21  "GcCDP_MaxCellTemp_C"
  Bus Selector/5 -> ACChrgPermit/5(GeVDP_VcuFalutLvl_enum)  "<GeVDP_VcuFalutLvl_enum>"
  Bus Selector/6 -> ACChrgPermit/6(GcCDP_MinCellTemp_C)  "<GcCDP_MinCellTemp_C>"
  Bus Selector/7 -> ACChrgPermit/7(GcCDP_MaxCellTemp_C)  "<GcCDP_MaxCellTemp_C>"
  GeODP_ObcChrgSt_enum/1 -> Bus Creator/22  "GeODP_ObcChrgSt_enum"
  Bus Selector/8 -> ACChrgPermit/8(GeODP_ObcChrgSt_enum)  "<GeODP_ObcChrgSt_enum>"
  ACChrgPermit/2(LbACC_ACChrgPrmt_flg) -> ACChrgCtl/2(LbACC_ACChrgPrmt_flg)
  Bus Selector6/1 -> PreHeatCtl/1(GcCDP_MinCellTemp_C)  "<GcCDP_MinCellTemp_C>"
  GeVDP_PreThmVcuPmt_enum/1 -> Bus Creator/23  "GeVDP_PreThmVcuPmt_enum"
  GeVDP_PreThmEna_enum/1 -> Bus Creator/24  "GeVDP_PreThmEna_enum"
  Bus Selector6/2 -> PreHeatCtl/2(GeMSM_BMUState_enum)  "<GeMSM_BMUState_enum>"
  Bus Selector6/3 -> PreHeatCtl/3(GbWSM_ACWkUpPrs_flg)  "<GbWSM_ACWkUpPrs_flg>"
  Bus Selector6/4 -> PreHeatCtl/4(GbODP_ACChrgAllow_flg)  "<GbODP_ACChrgAllow_flg>"
  Bus Selector6/5 -> PreHeatCtl/5(GcSOC_DispSOC_pct)  "<GcSOC_DispSOC_pct>"
  Bus Selector6/6 -> PreHeatCtl/6(GeVDP_VcuFalutLvl_enum)  "<GeVDP_VcuFalutLvl_enum>"
  Bus Selector6/7 -> PreHeatCtl/7(GeVDP_PreThmVcuPmt_enum)  "<GeVDP_PreThmVcuPmt_enum>"
  Bus Selector6/8 -> PreHeatCtl/8(GeODP_ObcChrgSt_enum)  "<GeODP_ObcChrgSt_enum>"
  Bus Selector6/9 -> PreHeatCtl/9(GeCTC_CtrCtlState_enum)  "<GeCTC_CtrCtlState_enum>"
  Bus Selector6/10 -> PreHeatCtl/10(GcHDP_PackVolt_V)  "<GcHDP_PackVolt_V>"
  PreHeatCtl/2(GbACC_PreThmRqst_flg) -> GbACC_PreThmRqst_flg/1
  PreHeatCtl/1(GbACC_PreHeatPrmt_flg) -> ACChrgPermit/16(GbACC_PreHeatPrmt_flg), GbACC_PreHeatPrmt_flg/1
  PreHeatCtl/3(GbACC_PreThmObcChrgCmd_flg) -> GbACC_PreThmObcChrgCmd_flg/1
  PreHeatCtl/4(GcACC_PreThmCrntRqst_A) -> GcACC_PreThmCrntRqst_A/1
  PreHeatCtl/5(GcACC_PreThmVoltRqst_V) -> GcACC_PreThmVoltRqst_V/1
  GcHDP_PackCrnt_A/1 -> Bus Creator/25  "GcHDP_PackCrnt_A"
  GcSOC_PackSOC_pct/1 -> Bus Creator/26  "GcSOC_PackSOC_pct"
  GeODP_ObcCcSt_enum/1 -> Bus Creator/27  "GeODP_ObcCcSt_enum"
  GcODP_ObcCpDuty_numb/1 -> Bus Creator/28  "GcODP_ObcCpDuty_numb"
  Bus Selector7/1 -> ACChrgRemainingTime/2(GcHDP_PackCrnt_A)  "<GcHDP_PackCrnt_A>"
  Bus Selector7/2 -> ACChrgRemainingTime/3(GcHDP_PackVolt_V)  "<GcHDP_PackVolt_V>"
  Bus Selector7/3 -> ACChrgRemainingTime/4(GeODP_ObcCcSt_enum)  "<GeODP_ObcCcSt_enum>"
  Bus Selector7/4 -> ACChrgRemainingTime/5(GcODP_ObcCpDuty_numb)  "<GcODP_ObcCpDuty_numb>"
  Bus Selector7/5 -> ACChrgRemainingTime/6(GeODP_ObcElecLck_enum)  "<GeODP_ObcElecLck_enum>"
  Bus Selector7/6 -> ACChrgRemainingTime/7(GcVDP_ChrgLdReq_numb)  "<GcVDP_ChrgLdReq_numb>"
  Bus Selector7/7 -> ACChrgRemainingTime/8(GeODP_ObcChrgSt_enum)  "<GeODP_ObcChrgSt_enum>"
  GcODP_MaxPwrObcChrg_W/1 -> Bus Creator/29  "GcODP_MaxPwrObcChrg_W"
  Bus Selector7/8 -> ACChrgRemainingTime/9(GcODP_MaxPwrObcChrg_W)  "<GcODP_MaxPwrObcChrg_W>"
  ACChrgCtl/9(GbACC_ChrgSt2StepChrg_flg) -> GbACC_ChrgSt2StepChrg_flg/1
  GbFTC_OpenContactor_flg/1 -> Bus Creator/30  "GbFTC_OpenContactor_flg"
  GbFTC_PowerDown_flg/1 -> Bus Creator/31  "GbFTC_PowerDown_flg"
  Bus Selector6/11 -> PreHeatCtl/11(GbFTC_OpenContactor_flg)  "<GbFTC_OpenContactor_flg>"
  Bus Selector6/12 -> PreHeatCtl/12(GbFTC_PowerDown_flg)  "<GbFTC_PowerDown_flg>"
  Bus Selector/9 -> ACChrgPermit/9(GbFTC_OpenContactor_flg)  "<GbFTC_OpenContactor_flg>"
  Bus Selector/10 -> ACChrgPermit/10(GbFTC_PowerDown_flg)  "<GbFTC_PowerDown_flg>"
  GbVDP_VcuChrgDisable_flg/1 -> Bus Creator/32  "GbVDP_VcuChrgDisable_flg"
  Bus Selector/11 -> ACChrgPermit/11(GbVDP_VcuChrgDisable_flg)  "<GbVDP_VcuChrgDisable_flg>"
  Bus Selector1/13 -> ACChrgCtl/15(GcSOC_DispSOC_pct)  "<GcSOC_DispSOC_pct>"
  Bus Selector/12 -> ACChrgPermit/12(GcODP_ObcFaultLvl_numb)  "<GcODP_ObcFaultLvl_numb>"
  Bus Selector6/13 -> PreHeatCtl/13(GcODP_ObcFaultLvl_numb)  "<GcODP_ObcFaultLvl_numb>"
  Bus Selector6/14 -> PreHeatCtl/14(GeVDP_PreThmEna_enum)  "<GeVDP_PreThmEna_enum>"
  Bus Selector6/15 -> PreHeatCtl/15(GcODP_CurrObcChrg_A)  "<GcODP_CurrObcChrg_A>"
  GeODP_ObcCpSt_enum/1 -> Bus Creator/33  "GeODP_ObcCpSt_enum"
  Bus Selector1/14 -> ACChrgCtl/16(GeODP_ObcCpSt_enum)  "<GeODP_ObcCpSt_enum>"
  GeUDS_AreaSel_enum/1 -> Bus Creator/34  "GeUDS_AreaSel_enum"
  Bus Selector1/15 -> ACChrgCtl/17(GeUDS_AreaSel_enum)  "<GeUDS_AreaSel_enum>"
  GcUDS_FullChrgCutoffVolt_mV/1 -> Bus Creator/35  "GcUDS_FullChrgCutoffVolt_mV"
  Bus Selector1/16 -> ACChrgCtl/18(GcUDS_FullChrgCutoffVolt_mV)  "<GcUDS_FullChrgCutoffVolt_mV>"
  GcUDS_BatEnergy_kWh/1 -> Bus Creator/36  "GcUDS_BatEnergy_kWh"
  GeUDS_CapSel_enum/1 -> Bus Creator/37  "GeUDS_CapSel_enum"
  Bus Selector7/9 -> ACChrgRemainingTime/10(GcUDS_BatEnergy_kWh)  "<GcUDS_BatEnergy_kWh>"
  Bus Selector7/10 -> ACChrgRemainingTime/11(GeUDS_CapSel_enum)  "<GeUDS_CapSel_enum>"
  GeADP_RmPreThemalReq_enum/1 -> Bus Creator/38  "GeADP_RmPreThemalReq_enum"
  GcADP_RmPreThemalTime_min/1 -> Bus Creator/39  "GcADP_RmPreThemalTime_min"
  GbWSM_Kl15WkUpPrs_flg/1 -> Bus Creator/40  "GbWSM_Kl15WkUpPrs_flg"
  Bus Selector8/1 -> HoldTempCtl/1(GeMSM_BMUState_enum)  "<GeMSM_BMUState_enum>"
  Bus Selector8/2 -> HoldTempCtl/2(GbWSM_ACWkUpPrs_flg)  "<GbWSM_ACWkUpPrs_flg>"
  Bus Selector8/3 -> HoldTempCtl/3(GbODP_ACChrgAllow_flg)  "<GbODP_ACChrgAllow_flg>"
  Bus Selector8/4 -> HoldTempCtl/4(GcSOC_DispSOC_pct)  "<GcSOC_DispSOC_pct>"
  Bus Selector8/5 -> HoldTempCtl/5(GeVDP_VcuFalutLvl_enum)  "<GeVDP_VcuFalutLvl_enum>"
  Bus Selector8/6 -> HoldTempCtl/6(GeVDP_PreThmVcuPmt_enum)  "<GeVDP_PreThmVcuPmt_enum>"
  Bus Selector8/7 -> HoldTempCtl/7(GeODP_ObcChrgSt_enum)  "<GeODP_ObcChrgSt_enum>"
  Bus Selector8/8 -> HoldTempCtl/8(GeCTC_CtrCtlState_enum)  "<GeCTC_CtrCtlState_enum>"
  Bus Selector8/9 -> HoldTempCtl/9(GcHDP_PackVolt_V)  "<GcHDP_PackVolt_V>"
  Bus Selector8/10 -> HoldTempCtl/10(GbFTC_OpenContactor_flg)  "<GbFTC_OpenContactor_flg>"
  Bus Selector8/11 -> HoldTempCtl/11(GbFTC_PowerDown_flg)  "<GbFTC_PowerDown_flg>"
  Bus Selector8/12 -> HoldTempCtl/12(GcODP_ObcFaultLvl_numb)  "<GcODP_ObcFaultLvl_numb>"
  Bus Selector8/13 -> HoldTempCtl/13(GbWSM_Kl15WkUpPrs_flg)  "<GbWSM_Kl15WkUpPrs_flg>"
  Bus Selector8/14 -> HoldTempCtl/14(GeADP_RmPreThemalReq_enum)  "<GeADP_RmPreThemalReq_enum>"
  Bus Selector8/15 -> HoldTempCtl/15(GcADP_RmPreThemalTime_min)  "<GcADP_RmPreThemalTime_min>"
  HoldTempCtl/4(GcACC_HoldTempCrntRqst_A) -> GcACC_HoldTempCrntRqst_A/1
  HoldTempCtl/5(GcACC_HoldTempVoltRqst_V) -> GcACC_HoldTempVoltRqst_V/1
  HoldTempCtl/3(GbACC_HoldTempObcChrgCmd_flg) -> GbACC_HoldTempObcChrgCmd_flg/1
  HoldTempCtl/2(GbACC_HoldTempRqst_flg) -> GbACC_HoldTempRqst_flg/1
  HoldTempCtl/1(GbACC_HoldTempPrmt_flg) -> GbACC_HoldTempPrmt_flg/1
  GbADP_StopChgReq_flg/1 -> Bus Creator/41  "GbADP_StopChgReq_flg"
  Bus Selector/13 -> ACChrgPermit/13(GbADP_StopChgReq_flg)  "<GbADP_StopChgReq_flg>"
  Bus Selector7/11 -> ACChrgRemainingTime/12(GcSOC_DispSOC_pct)  "<GcSOC_DispSOC_pct>"
  Bus Selector6/16 -> PreHeatCtl/16(GbADP_StopChgReq_flg)  "<GbADP_StopChgReq_flg>"
  Bus Selector8/16 -> HoldTempCtl/16(GbADP_StopChgReq_flg)  "<GbADP_StopChgReq_flg>"
  Bus Selector7/12 -> ACChrgRemainingTime/13(GcCDP_MaxCellVolt_mV)  "<GcCDP_MaxCellVolt_mV>"
  Bus Selector7/13 -> ACChrgRemainingTime/14(GcUDS_FullChrgCutoffVolt_mV)  "<GcUDS_FullChrgCutoffVolt_mV>"
  Bus Selector6/17 -> PreHeatCtl/17(GbADP_ChrgStopActive_flg)  "<GbADP_ChrgStopActive_flg>"
  Bus Selector6/18 -> PreHeatCtl/18(GeUDS_AreaSel_enum)  "<GeUDS_AreaSel_enum>"
  Bus Selector8/17 -> HoldTempCtl/17(GbADP_ChrgStopActive_flg)  "<GbADP_ChrgStopActive_flg>"
  Bus Selector8/18 -> HoldTempCtl/18(GeUDS_AreaSel_enum)  "<GeUDS_AreaSel_enum>"
  Bus Selector/14 -> ACChrgPermit/14(GcHDP_PackVolt_V)  "<GcHDP_PackVolt_V>"
  GbFTC_InhACChrg_flg/1 -> Bus Creator/42  "GbFTC_InhACChrg_flg"
  Bus Selector6/19 -> PreHeatCtl/19(GbFTC_InhACChrg_flg)  "<GbFTC_InhACChrg_flg>"
  Bus Selector/15 -> ACChrgPermit/15(GbFTC_InhACChrg_flg)  "<GbFTC_InhACChrg_flg>"
  Bus Selector8/19 -> HoldTempCtl/19(GbFTC_InhACChrg_flg)  "<GbFTC_InhACChrg_flg>"

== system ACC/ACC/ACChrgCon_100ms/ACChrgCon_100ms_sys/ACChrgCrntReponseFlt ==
  GcODP_CurrObcChrg_A : Inport
  GeACC_ACChrgState_enum : Inport  Port=2
  GcACC_ACChrgCrntRqst_A : Inport  Port=3
  ACC_GbACC_ACChrgCrntFlt_flg : AIWAYS_Powertrain_BMS_lib/Signals/OverWrite  OverWrite_Value=CbACC_ACChrgCrntFltOvr_flg  OverWrite_flag=CbACC_ACChrgCrntFltOvrSwt_flg
  BMSDebounceStartZero : AIWAYS_Powertrain_BMS_lib/Debounce & Delay/BMSDebounceStartZero
  Constant1 : Constant  Value=CcACC_DiffACChrgCrnt_A
  Constant2 : Constant  Value=Enum_ACCACChrgState.Enum_ACCACChrgState_Chrg
  Constant3 : Constant  Value=Enum_ACCACChrgState.Enum_ACCACChrgState_StepChrg
  Constant4 : Constant  Value=CcACC_DiffACChrgCrntTi_ms
  Constant5 : Constant  Value=ACC_RUNTIME_MS
  Constant6 : Constant  Value=CcACC_DiffACChrgCrntTi_ms
  Constant7 : Constant  Value=ACC_RUNTIME_MS
  Data Type Conversion3 : DataTypeConversion
  DiffValue : AIWAYS_Powertrain_BMS_lib/Mathematical Functions/DiffValue
  Logical Operator : Logic  Operator=OR  AllPortsSameDT=off  OutDataTypeStr=boolean
  Logical Operator1 : Logic  AllPortsSameDT=off  OutDataTypeStr=boolean
  Relational Operator1 : RelationalOperator  Operator=>  OutDataTypeStr=boolean
  Relational Operator2 : RelationalOperator  Operator===  OutDataTypeStr=boolean
  Relational Operator3 : RelationalOperator  Operator===  OutDataTypeStr=boolean
  GbACC_ACChrgCrntFlt_flg : Outport
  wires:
  Data Type Conversion3/1 -> Relational Operator3/1, Relational Operator2/1
  Relational Operator1/1 -> Logical Operator1/2
  Logical Operator/1 -> Logical Operator1/1
  Relational Operator3/1 -> Logical Operator/2
  Relational Operator2/1 -> Logical Operator/1
  Constant3/1 -> Relational Operator3/2
  GeACC_ACChrgState_enum/1 -> Data Type Conversion3/1
  Constant2/1 -> Relational Operator2/2
  Constant1/1 -> Relational Operator1/2
  GcACC_ACChrgCrntRqst_A/1 -> DiffValue/1
  GcODP_CurrObcChrg_A/1 -> DiffValue/2
  DiffValue/1 -> Relational Operator1/1
  Logical Operator1/1 -> BMSDebounceStartZero/1
  Constant4/1 -> BMSDebounceStartZero/2
  Constant6/1 -> BMSDebounceStartZero/4
  Constant5/1 -> BMSDebounceStartZero/3
  Constant7/1 -> BMSDebounceStartZero/5
  ACC_GbACC_ACChrgCrntFlt_flg/1 -> GbACC_ACChrgCrntFlt_flg/1  "GbACC_ACChrgCrntFlt_flg"
  BMSDebounceStartZero/1 -> ACC_GbACC_ACChrgCrntFlt_flg/1
